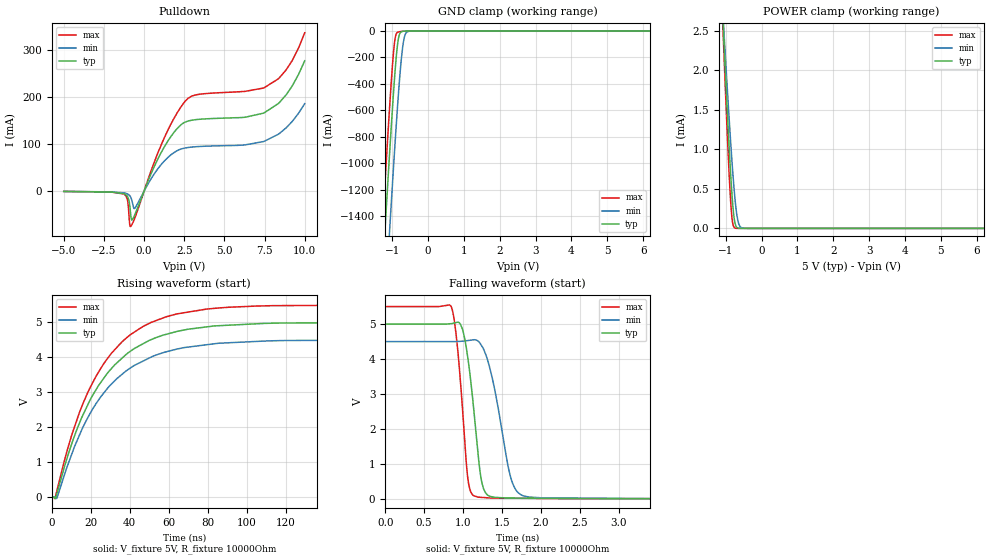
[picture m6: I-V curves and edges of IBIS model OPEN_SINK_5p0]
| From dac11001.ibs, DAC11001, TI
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|   OPEN_SINK_5p0
[Model]   OPEN_SINK_5p0
Model_type   Open_sink
Polarity   Non-Inverting
Vmeas = 2.5
Vref = 5
Cref = 2pF
Rref = 10000
|   typ   min   max
C_comp   0.835pF   0.812pF   0.843pF
[Voltage Range]   5   4.5   5.5
[Temperature Range]   25   125   -40
[Pullup Reference]   5   4.5   5.5
[Pulldown Reference]   0   0   0
[Power Clamp Reference]   5   4.5   5.5
[GND Clamp Reference]   0   0   0
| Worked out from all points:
|   slope of the pulldown table from 0 to 0.75 V, typ, clamps not added: 12.3 ohm
|   GND clamp passes 1 mA (typ) near -0.68 V on its own axis
|   POWER clamp passes 1 mA (typ) near -0.91 V on its own axis
|   falling waveform, V_fixture 5V, R_fixture 10000Ohm: 20-80 % time 143ps typ, 222ps min, 114ps max; typ from 5 V to 0.006 V
|   rising waveform, V_fixture 5V, R_fixture 10000Ohm: 20-80 % time 29.3ns typ, 29.8ns min, 28.5ns max; typ from 0.006 V to 5 V
[Pulldown]
|   Voltage   I(typ)   I(min)   I(max)
-5V       -486.9uA   -443.1uA   -440.4uA
-1.25V    -5.234mA   -3.5mA     -6.052mA
-1.025V   -11.65mA   -5.875mA   -19.84mA
-845mV    -45.07mA   -11.86mA   -75.22mA
-770mV    -61.28mA   -18.4mA    -71.8mA
-575mV    -49.92mA   -36.31mA   -57.09mA
1.06V     81.95mA    56.47mA    97.94mA
2.53V     146.6mA    91.77mA    190.1mA
3.37V     152.7mA    94.95mA    205.8mA
7.48V     166.7mA    106.2mA    220.1mA
8.845V    205mA      134.8mA    258mA
10V       277.4mA    186.2mA    336.8mA
[GND Clamp]
|   Voltage   I(typ)   I(min)   I(max)
-5V       -20.14A    -20.68A    -19.83A
-1.43V    -2.558A    -3.149A    -2.204A
-1.25V    -1.71A     -2.303A    -1.354A
-1.235V   -1.64A     -2.233A    -1.284A
-1.175V   -1.364A    -1.956A    -1.009A
-1.085V   -959.2mA   -1.546A    -609.9mA
-950mV    -398mA     -953.9mA   -112.6mA
-845mV    -81.3mA    -529.9mA   -8.172mA
-755mV    -5.965mA   -226.2mA   -3.349mA
-695mV    -1.264mA   -88.24mA   -1.713mA
-530mV    -35.72uA   -1.253mA   -60.62uA
10V       0A         0A         0A
[POWER Clamp]
|   Voltage   I(typ)   I(min)   I(max)
-5V       44.14mA    36.55mA    51.17mA
-1.1V     2.805mA    2.855mA    2.736mA
-1.04V    2.224mA    2.381mA    2.055mA
-920mV    1.126mA    1.473mA    793.4uA
-860mV    641.8uA    1.05mA     298.9uA
-815mV    341.8uA    757.5uA    82.25uA
-770mV    134.4uA    496.6uA    12.85uA
-740mV    58.52uA    348uA      3.168uA
-695mV    13.03uA    176.2uA    354.3nA
-650mV    2.499uA    72.81uA    26.1nA
-530mV    10.46nA    3.305uA    0A
10V       0A         0A         0A
[Ramp]
R_load = 10000
|   typ   min   max
dV/dt_r   2.99669/2.91237e-08   2.69589/2.9822e-08   3.29683/2.84814e-08
dV/dt_f   2.99669/1.42228e-10   2.69589/2.21006e-10   3.29683/1.13784e-10
[Falling Waveform]
V_fixture = 5V
V_fixture_min = 4.5V
V_fixture_max = 5.5V
R_fixture = 10000Ohm
C_fixture = 0F
|   Time   V(typ)   V(min)   V(max)
0s        5V         4.5V       5.5V
844.7ps   5.012V     4.5V       5.51V
990.1ps   4.865V     4.51V      2.638V
1.056ns   4.094V     4.527V     665.7mV
1.121ns   2.896V     4.547V     118.2mV
1.226ns   645.2mV    4.42V      44.11mV
1.31ns    116.2mV    4.003V     31.28mV
1.667ns   23.39mV    292mV      18.8mV
2.347ns   11.43mV    23.9mV     5.891mV
3.5us     5.521mV    6.852mV    5.276mV
[Rising Waveform]
V_fixture = 5V
V_fixture_min = 4.5V
V_fixture_max = 5.5V
R_fixture = 10000Ohm
C_fixture = 0F
|   Time   V(typ)   V(min)   V(max)
0s        5.521mV    6.852mV    5.276mV
1.571ns   -33.25mV   -4.441mV   -44.63mV
2.692ns   102.3mV    -26.37mV   188mV
10.49ns   1.559V     1.259V     1.81V
18.21ns   2.606V     2.241V     2.955V
26.33ns   3.371V     2.951V     3.787V
35.98ns   3.971V     3.509V     4.439V
58.73ns   4.659V     4.158V     5.161V
104.8ns   4.959V     4.454V     5.468V
3.5us     5V         4.5V       5.5V
